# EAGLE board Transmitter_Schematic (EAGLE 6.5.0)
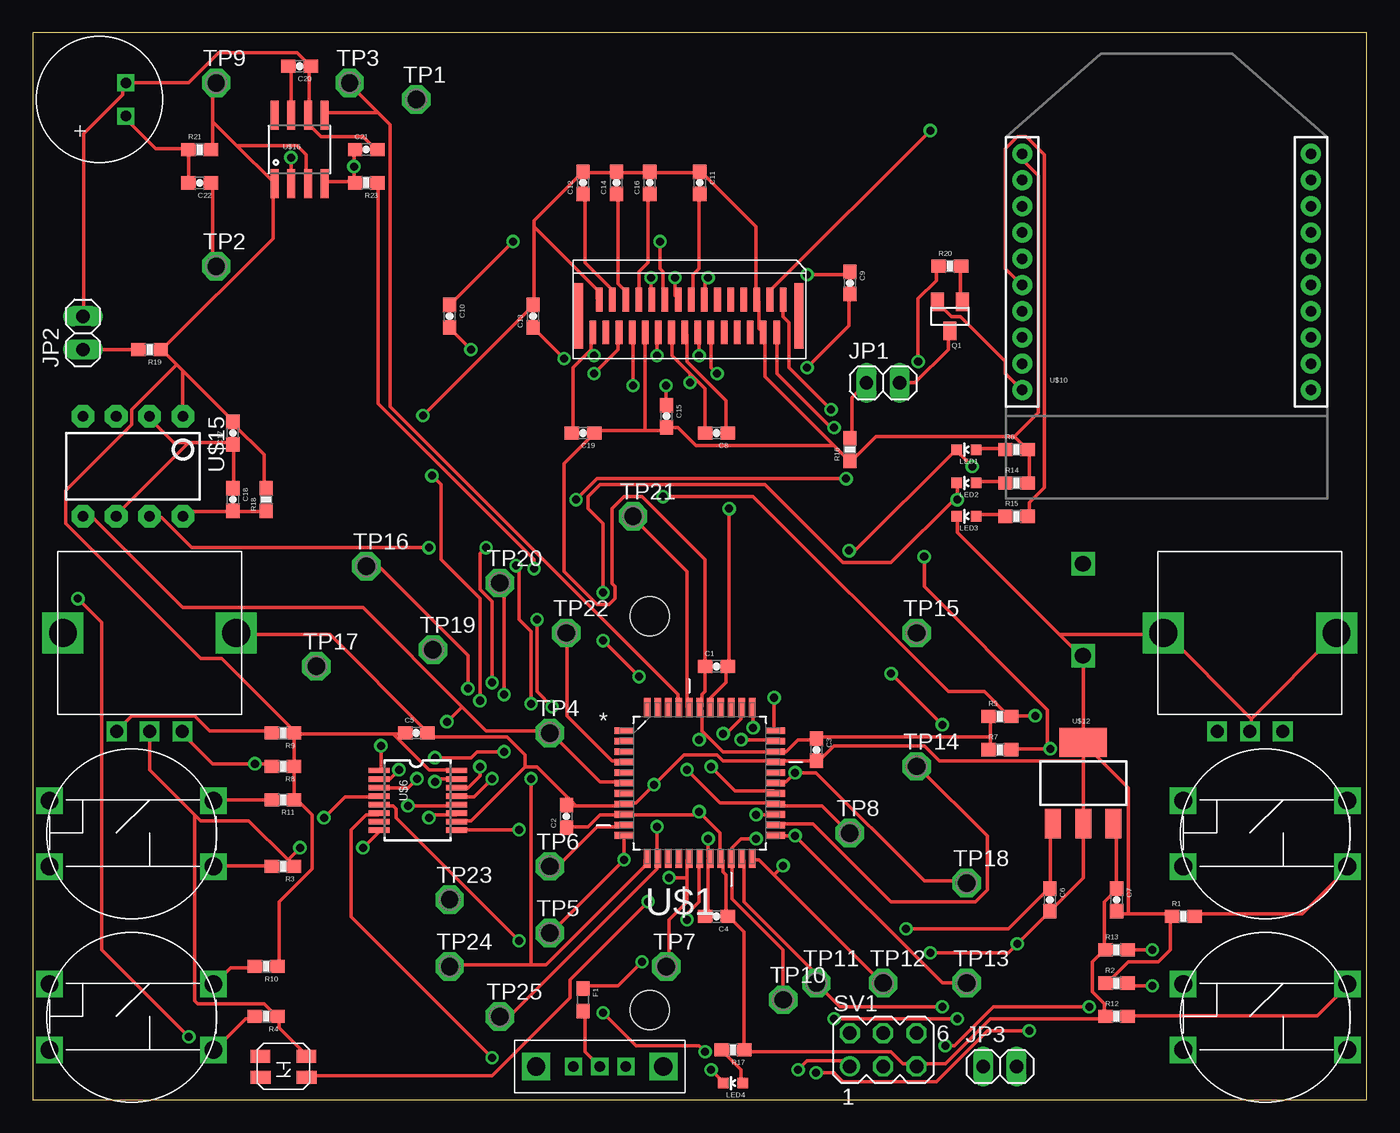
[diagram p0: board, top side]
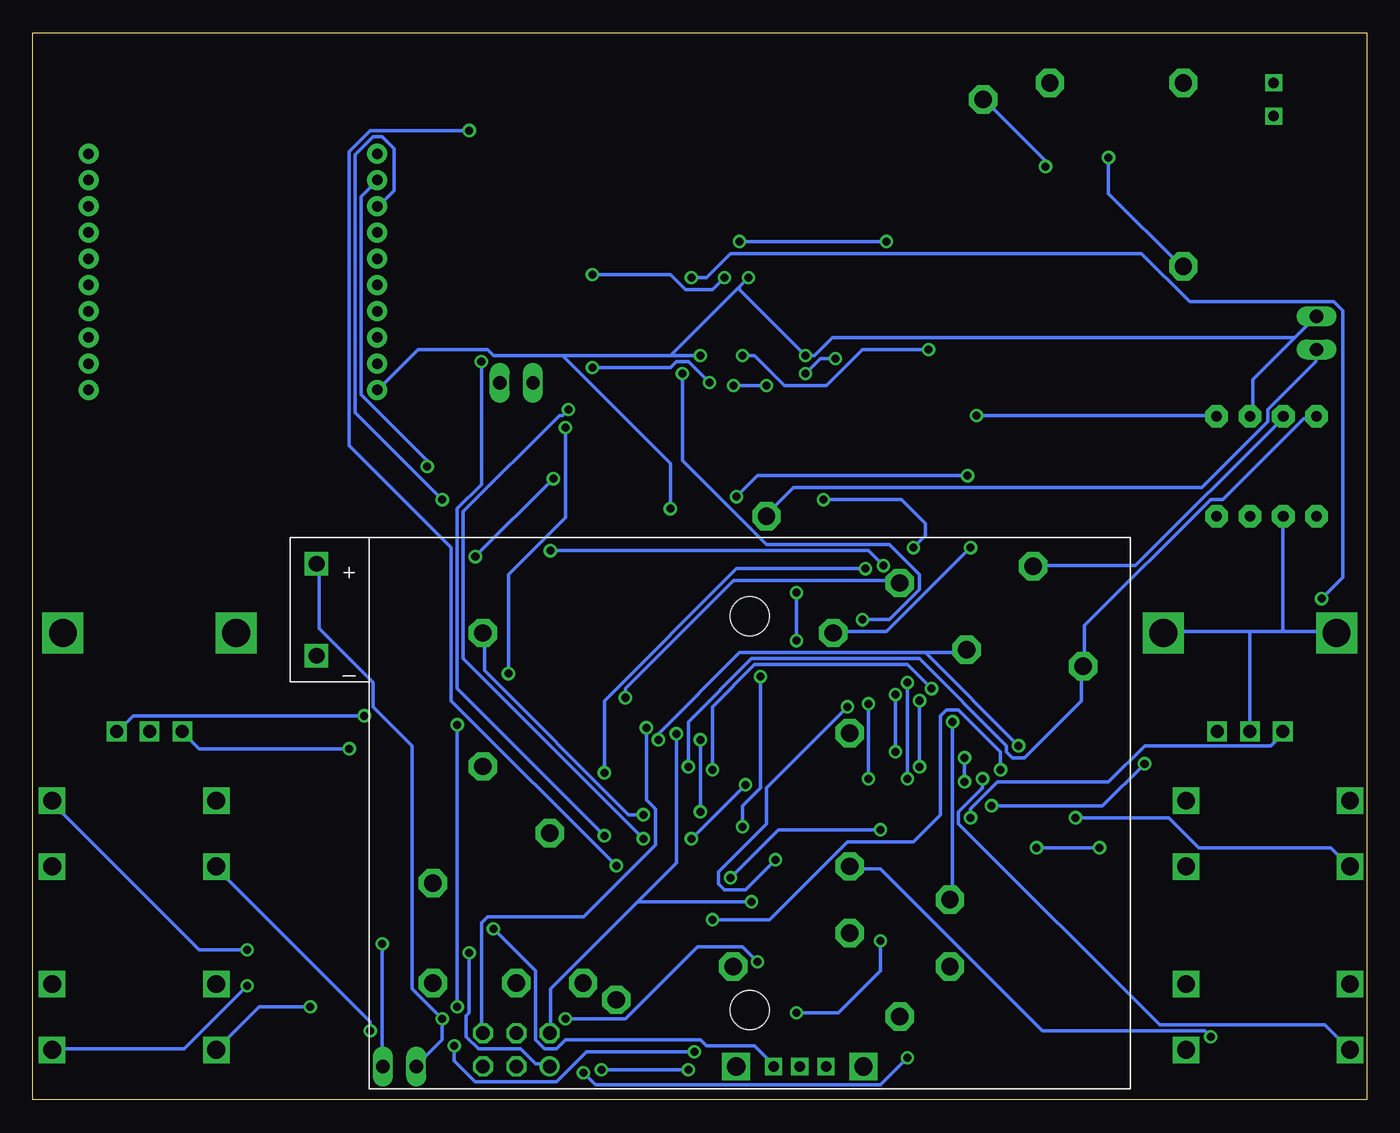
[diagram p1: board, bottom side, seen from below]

Size 101.6 x 81.28 mm. Coordinates in mm from the lower left corner, seen from the top.
Outline: 0,0 101.6,0 101.6,81.28 0,81.28 0,0
Copper layers (1*16): Top 0.035mm / dielectric 1.5mm / Bottom 0.035mm
Design rules "default": minimum track width 10mil, minimum drill 24mil, track to track 8mil, track to pad 8mil, pad to pad 8mil, via to via 8mil, smd to smd 8mil, copper to edge 40mil, drill to drill 8mil, minimum pad ring 10mil, minimum via ring 8mil, stop-mask expansion 4mil, vias tented up to drill 0mil, thermal gap 10mil

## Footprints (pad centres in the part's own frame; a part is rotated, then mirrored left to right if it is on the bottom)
0603-CAP = smd 1.1 x 1: 1 -0.85,0; 2 0.85,0
0603 = smd 1.1 x 1: 1 -0.85,0; 2 0.85,0
1X02 = drill 1.016 long: 1 -1.27,0; 2 1.27,0
LED-0603 = smd 0.8 x 0.8: A 0,-0.75; C 0,0.75
SOT23 = smd 1 x 1.4: 1 -0.95,-1.1; 2 0.95,-1.1; 3 0,1.1
0603-RES = smd 1.1 x 1: 1 -0.85,0; 2 0.85,0
MA03-2 = drill 1.016: 1 -2.54,-1.27 | drill 1.016 octagon: 2 -2.54,1.27; 3 0,-1.27; 4 0,1.27; 5 2.54,-1.27; 6 2.54,1.27
SPARKFUN_TAC_BUTTONS = drill 1.346 square: 1 0,5.004; 2 12.497,5.004; 3 0,0; 4 12.497,0
P1-13 = drill 1.321 pad 2.159 octagon: TP 0,0
QFP80P1200X1200X120-44N = smd 1.473 x 0.508: 1 -5.74,3.988; 2 -5.74,3.2; 3 -5.74,2.388; 4 -5.74,1.6; 5 -5.74,0.787; 6 -5.74,0; 7 -5.74,-0.787; 8 -5.74,-1.6; 9 -5.74,-2.388; 10 -5.74,-3.2; 11 -5.74,-3.988; 23 5.74,-3.988; 24 5.74,-3.2; 25 5.74,-2.388; 26 5.74,-1.6; 27 5.74,-0.787; 28 5.74,0; 29 5.74,0.787; 30 5.74,1.6; 31 5.74,2.388; 32 5.74,3.2; 33 5.74,3.988 | smd 0.508 x 1.473: 12 -3.988,-5.74; 13 -3.2,-5.74; 14 -2.388,-5.74; 15 -1.6,-5.74; 16 -0.787,-5.74; 17 0,-5.74; 18 0.787,-5.74; 19 1.6,-5.74; 20 2.388,-5.74; 21 3.2,-5.74; 22 3.988,-5.74; 34 3.988,5.74; 35 3.2,5.74; 36 2.388,5.74; 37 1.6,5.74; 38 0.787,5.74; 39 0,5.74; 40 -0.787,5.74; 41 -1.6,5.74; 42 -2.388,5.74; 43 -3.2,5.74; 44 -3.988,5.74
TSSOP16 = smd 0.4 x 1.6: 1 -2.225,-2.85; 2 -1.575,-2.85; 3 -0.925,-2.85; 4 -0.275,-2.85; 5 0.375,-2.85; 6 1.025,-2.85; 7 1.675,-2.85; 8 2.325,-2.85; 9 2.325,3.05; 10 1.675,3.05; 11 1.025,3.05; 12 0.375,3.05; 13 -0.275,3.05; 14 -0.925,3.05; 15 -1.575,3.05; 16 -2.225,3.05
MICRO_TAC_BUTTONS = smd 1.524 x 1: 1 0.75,2.1; 3 4.25,2.1 | smd 1.5 x 1: 2 0.75,0.5; 4 4.25,0.5
EVE_GE1F2012B = drill 2.1 square: @GND1 -6.6,0; @GND2 6.6,0 | drill 1 square: A -2.5,-7.5; B 2.5,-7.5; GND 0,-7.5
XBEE-1 = drill 0.8 pad 1.524: 1 -11,20; 2 -11,18; 3 -11,16; 4 -11,14; 5 -11,12; 6 -11,10; 7 -11,8; 8 -11,6; 9 -11,4; 10 -11,2; 11 11,2; 12 11,4; 13 11,6; 14 11,8; 15 11,10; 16 11,12; 17 11,14; 18 11,16; 19 11,18; 20 11,20
LCD_CONNECTOR = smd 0.5 x 1.8: 1 0,0; 2 -0.5,-2.5; 3 -1,0; 4 -1.5,-2.5; 5 -2,0; 6 -2.5,-2.5; 7 -3,0; 8 -3.5,-2.5; 9 -4,0; 10 -4.5,-2.5; 11 -5,0; 12 -5.5,-2.5; 13 -6,0; 14 -6.5,-2.5; 15 -7,0; 16 -7.5,-2.5; 17 -8,0; 18 -8.5,-2.5; 19 -9,0; 20 -9.5,-2.5; 21 -10,0; 22 -10.5,-2.5; 23 -11,0; 24 -11.5,-2.5; 25 -12,0; 26 -12.5,-2.5; 27 -13,0; 28 -13.5,-2.5; 29 -14,0; 30 -14.5,-2.5 | smd 0.7 x 5: 31 1.2,-1.25; 32 -15.6,-1.25
SOT223 = smd 1.219 x 2.235: 1 -2.311,-3.099; 2 0,-3.099; 3 2.311,-3.099 | smd 3.6 x 2.2: 4 0,3.099
3XAA_BATT_HOLDER = drill 1.2 square: + 33,-4; - 33,3 | hole 3: 0,30; 0,0
SWITCH_SLIDE = drill 0.8 square: 1 -2,0; 2 0,0; 3 2,0 | drill 1.41 square: P$4 4.85,0 | drill 1.4 square: P$5 -4.85,0
DIP08 = drill 0.813 pad 1.727 octagon: 1 -3.81,-3.81; 2 -1.27,-3.81; 3 1.27,-3.81; 4 3.81,-3.81; 5 3.81,3.81; 6 1.27,3.81; 7 -1.27,3.81; 8 -3.81,3.81
SOIC8 = smd 0.61 x 2.21: 1 -1.905,-2.616; 2 -0.635,-2.616; 3 0.635,-2.616; 4 1.905,-2.616; 5 1.905,2.616; 6 0.635,2.616; 7 -0.635,2.616; 8 -1.905,2.616
CMA-4544PF = drill 0.8 square: GND 2,1.27; OUT 2,-1.27

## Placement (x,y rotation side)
C1  0.1uF  [0603-CAP]  52.07,33.02 0 top
C2  0.1uF  [0603-CAP]  40.64,21.59 90 top
C3  0.1uF  [0603-CAP]  59.69,26.67 270 top
C4  0.1uF  [0603-CAP]  52.07,13.97 180 top
C5  0.1uF  [0603-CAP]  29.21,27.94 0 top
C6  0.1uF  [0603-CAP]  77.47,15.24 270 top
C7  10uF  [0603-CAP]  82.55,15.24 270 top
C8  0.1uF  [0603-CAP]  52.07,50.8 180 top
C9  0.1uF  [0603-CAP]  62.23,62.23 270 top
C10  0.1uF  [0603-CAP]  31.75,59.69 270 top
C11  0.1uF  [0603-CAP]  50.8,69.85 270 top
C12  0.1uF  [0603-CAP]  41.91,69.85 90 top
C13  0.1uF  [0603-CAP]  38.1,59.69 90 top
C14  0.1uF  [0603-CAP]  44.45,69.85 90 top
C15  0.1uF  [0603-CAP]  48.26,52.07 270 top
C16  0.1uF  [0603-CAP]  46.99,69.85 90 top
C17  0.1uF  [0603-CAP]  15.24,50.8 90 top
C18  0.33pF  [0603-CAP]  15.24,45.72 270 top
C19  0.1uF  [0603-CAP]  41.91,50.8 180 top
C20  0.1uF  [0603-CAP]  20.32,78.74 180 top
C21  0.1uF  [0603-CAP]  25.4,72.39 0 top
C22  0.1uF  [0603-CAP]  12.7,69.85 180 top
F1  PTC0603  [0603]  41.91,7.62 270 top
JP1  [1X02]  64.77,54.61 0 top
JP2  [1X02]  3.81,58.42 90 top
JP3  [1X02]  73.66,2.54 0 top
LED1  [LED-0603]  71.12,49.53 90 top
LED2  [LED-0603]  71.12,46.99 90 top
LED3  [LED-0603]  71.12,44.45 90 top
LED4  [LED-0603]  53.34,1.27 90 top
Q1  MMBT5088  [SOT23]  69.85,59.69 180 top
R1  10K  [0603-RES]  87.63,13.97 0 top
R2  10K  [0603-RES]  82.55,8.89 0 top
R3  10K  [0603-RES]  19.05,17.78 180 top
R4  10K  [0603-RES]  17.78,6.35 180 top
R5  10K  [0603-RES]  73.66,29.21 0 top
R6  1K  [0603-RES]  74.93,49.53 0 top
R7  10K  [0603-RES]  73.66,26.67 0 top
R8  10K  [0603-RES]  19.05,25.4 180 top
R9  10K  [0603-RES]  19.05,27.94 180 top
R10  4.7K  [0603-RES]  17.78,10.16 180 top
R11  4.7K  [0603-RES]  19.05,22.86 180 top
R12  4.7K  [0603-RES]  82.55,6.35 0 top
R13  4.7K  [0603-RES]  82.55,11.43 0 top
R14  1K  [0603-RES]  74.93,46.99 0 top
R15  1K  [0603-RES]  74.93,44.45 0 top
R16  100  [0603-RES]  62.23,49.53 90 top
R17  1.5K  [0603-RES]  53.34,3.81 180 top
R18  200K  [0603-RES]  17.78,45.72 90 top
R19  10K  [0603-RES]  8.89,57.15 180 top
R20  100  [0603-RES]  69.85,63.5 0 top
R21  100  [0603-RES]  12.7,72.39 0 top
R23  100  [0603-RES]  25.4,69.85 180 top
SV1  [MA03-2]  64.77,3.81 0 top
SW0  SPARKFUN_TAC_BUTTONS  [SPARKFUN_TAC_BUTTONS]  1.27,3.81 0 top
SW1  SPARKFUN_TAC_BUTTONS  [SPARKFUN_TAC_BUTTONS]  1.27,17.78 0 top
SW2  SPARKFUN_TAC_BUTTONS  [SPARKFUN_TAC_BUTTONS]  87.63,3.81 0 top
SW3  SPARKFUN_TAC_BUTTONS  [SPARKFUN_TAC_BUTTONS]  87.63,17.78 0 top
TP1  TPPAD1-13  [P1-13]  29.21,76.2 0 top
TP2  TPPAD1-13  [P1-13]  13.97,63.5 0 top
TP3  TPPAD1-13  [P1-13]  24.13,77.47 0 top
TP4  TPPAD1-13  [P1-13]  39.37,27.94 0 top
TP5  TPPAD1-13  [P1-13]  39.37,12.7 0 top
TP6  TPPAD1-13  [P1-13]  39.37,17.78 0 top
TP7  TPPAD1-13  [P1-13]  48.26,10.16 0 top
TP8  TPPAD1-13  [P1-13]  62.23,20.32 0 top
TP9  TPPAD1-13  [P1-13]  13.97,77.47 0 top
TP10  TPPAD1-13  [P1-13]  57.15,7.62 0 top
TP11  TPPAD1-13  [P1-13]  59.69,8.89 0 top
TP12  TPPAD1-13  [P1-13]  64.77,8.89 0 top
TP13  TPPAD1-13  [P1-13]  71.12,8.89 0 top
TP14  TPPAD1-13  [P1-13]  67.31,25.4 0 top
TP15  TPPAD1-13  [P1-13]  67.31,35.56 0 top
TP16  TPPAD1-13  [P1-13]  25.4,40.64 0 top
TP17  TPPAD1-13  [P1-13]  21.59,33.02 0 top
TP18  TPPAD1-13  [P1-13]  71.12,16.51 0 top
TP19  TPPAD1-13  [P1-13]  30.48,34.29 0 top
TP20  TPPAD1-13  [P1-13]  35.56,39.37 0 top
TP21  TPPAD1-13  [P1-13]  45.72,44.45 0 top
TP22  TPPAD1-13  [P1-13]  40.64,35.56 0 top
TP23  TPPAD1-13  [P1-13]  31.75,15.24 0 top
TP24  TPPAD1-13  [P1-13]  31.75,10.16 0 top
TP25  TPPAD1-13  [P1-13]  35.56,6.35 0 top
U$1  ATXMEGA32A4UTQFP44  [QFP80P1200X1200X120-44N]  50.8,24.13 0 top
U$6  8B_SHIFT_REG  [TSSOP16]  29.21,22.86 270 top
U$7  MICRO_TAC_BUTTONS  [MICRO_TAC_BUTTONS]  21.59,3.81 180 top
U$8  ENCODER  [EVE_GE1F2012B]  8.89,35.56 0 top
U$9  ENCODER  [EVE_GE1F2012B]  92.71,35.56 0 top
U$10  XBEE-1B1  [XBEE-1]  86.36,52.07 0 top
U$11  LCD_CONNECTOR  [LCD_CONNECTOR]  57.15,60.96 0 top
U$12  3.3V_REG_LDO  [SOT223]  80.01,24.13 0 top
U$13  3XAA_BATT_HOLDER  [3XAA_BATT_HOLDER]  46.99,36.83 180 bottom
U$14  SWITCH_SLIDE  [SWITCH_SLIDE]  43.18,2.54 0 top
U$15  FREQUENCY_DIVIDER  [DIP08]  7.62,48.26 180 top
U$16  LM4875  [SOIC8]  20.32,72.39 0 top
U$17  MICROPHONE  [CMA-4544PF]  5.08,76.2 0 top

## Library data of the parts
C1-C22 = SparkFun-Capacitors
F1 = SparkFun-PowerIC
JP1-JP3 = pinhead
LED1-LED4 = SparkFun-LED
Q1 = SparkFun-DiscreteSemi; PROD_ID: TRANS-11160
R1-R21 R23 = SparkFun-Resistors
SV1 = con-lstb; OC_FARNELL: unknown; OC_NEWARK: unknown
SW0 SW1-SW3 U$1 U$6-U$9 U$11-U$17 = TuansLib
TP1-TP25 = testpad
U$10 = SparkFun-RF

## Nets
3.3V: C1.1 C2.1 C3.1 C4.1 C5.1 C7.1 C11.1 C12.2 C13.2 C14.2 C15.2 C16.2 C17.2 C19.1 R5.1 R6.2 R7.1 R8.1 R9.1 R10.1 R11.1 R12.1 R13.1 R14.2 R16.1 R17.1 R18.2 R19.1 R21.2 SV1.5 TP9.TP U$1.9 U$1.19 U$1.31 U$1.39 U$6.16 U$10.1 U$11.4 U$11.5 U$11.22 U$11.29 U$12.3 U$15.1 U$16.1 U$16.3
AUD_IN: TP3.TP U$1.41 U$16.5
AUD_VOL: R23.1 TP18.TP U$1.28
FQD_AUDIO: TP4.TP TP23.TP U$1.6 U$15.5
FQD_RST: TP22.TP U$1.4 U$15.7
GND: C1.2 C2.2 C3.2 C4.2 C5.2 C6.2 C7.2 C17.1 C18.1 C19.2 C20.1 C21.2 JP2.2 JP3.2 LED3.C LED4.C Q1.2 R1.1 R2.1 R3.1 R4.1 SV1.1 U$1.8 U$1.18 U$1.30 U$1.38 U$6.8 U$6.10 U$7.2 U$8.@GND1 U$8.@GND2 U$8.GND U$9.@GND1 U$9.@GND2 U$9.GND U$10.10 U$11.14 U$11.21 U$11.30 U$12.2 U$12.4 U$13.- U$15.2 U$15.6 U$16.6 U$17.GND
LCD_LIGHT: R20.1 TP13.TP U$1.23
LCD_RST: TP11.TP U$1.21 U$11.2
LCD_SIG-SEL: TP12.TP U$1.22 U$11.3
LCD_SS: TP10.TP U$1.20 U$11.1
MIC_IN: C22.1 TP2.TP U$16.2
N$1: R2.2 SW2.4
N$2: C6.1 U$12.1 U$14.3
N$4: C8.1 U$11.16
N$5: C8.2 C9.2 U$11.18
N$6: R3.2 SW1.4
N$7: R4.2 SW0.4
N$8: R1.2 SW3.4
N$9: R5.2 U$6.14 U$9.B
N$10: C9.1 U$11.17
N$11: R9.2 U$6.11 U$8.A
N$12: R8.2 U$6.12 U$8.B
N$13: R7.2 U$6.13 U$9.A
N$14: C10.2 U$11.20
N$15: R10.2 SW0.2
N$16: R11.2 SW1.2
N$17: R12.2 SW2.2
N$18: R13.2 SW3.2
N$19: C10.1 U$11.19
N$20: C12.1 U$11.27
N$21: C13.1 U$11.26
N$22: C14.1 U$11.25
N$23: C15.1 U$11.24
N$24: C16.1 U$11.23
N$25: JP1.1 R16.2
N$26: C11.2 U$11.15
N$27: JP1.2 Q1.3
N$28: F1.2 U$14.2
N$29: LED1.A R6.1
N$30: LED2.A R14.1
N$31: LED3.A R15.1
N$32: LED4.A R17.2
N$33: Q1.1 R20.2
N$34: C22.2 R21.1 U$17.OUT
N$35: C21.1 R23.2 TP1.TP U$16.4
N$37: C20.2 U$16.7
N$40: C18.2 R18.1 U$15.8
PDI: SV1.6 U$1.34
PWR_RAW: F1.1 JP3.1 U$13.+
RST/PDI_CLK: SV1.2 U$1.35 U$7.1
SHIFT_LATCH: TP20.TP U$1.33 U$6.15
SHIFT_LOAD: TP19.TP U$1.32 U$6.1
SPIC_MISO: TP7.TP U$1.16 U$6.9
SPIC_MOSI: U$1.15
SPIC_SCK: U$1.17 U$6.2
SPIC_SS: U$1.14
SPID_MISO: TP8.TP TP16.TP U$1.26 U$15.3
SPID_MOSI: TP15.TP U$1.25
SPID_SCK: TP17.TP U$1.27 U$15.4
SPID_SS: TP14.TP U$1.24
SW0: SW0.3 U$6.3
SW1: SW1.3 U$6.4
SW2: SW2.3 U$6.5
SW3: SW3.3 U$6.6
TEMP_SENSOR: JP2.1 R19.2 TP21.TP U$1.40
TWIC_SCL: TP5.TP U$1.11 U$11.12
TWIC_SDA: TP6.TP U$1.10 U$11.13
USART_RXC0: LED1.C TP24.TP U$1.12 U$10.2
USART_TXC0: LED2.C TP25.TP U$1.13 U$10.3
XBEE_RSSI: R15.2 U$10.6

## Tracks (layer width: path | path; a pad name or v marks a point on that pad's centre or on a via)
3.3V  (via drill 0.61)
  Top 0.254: 72.92,27.66 72.92,29.03 R5.1 | 72.92,27.66 72.92,26.75 R7.1 | 72.92,27.66 59.89,27.66 C3.1 59.66,27.43 58.29,27.43 57.38,26.52 U$1.31 52.58,26.52 51.21,27.89 | 51.21,27.89 50.98,28.12 50.98,29.72 U$1.39 50.98,29.95 50.98,30.86 51.21,31.09 51.21,32.92 C1.1 51.21,33.15 51.21,41.15 46.41,45.95 45.03,45.95 44.12,45.03 44.12,39.32 44.35,39.09 44.35,38.18 43.89,37.72 42.98,37.72 40.46,40.23 40.46,48.46 42.75,50.75 C19.1 42.98,50.98 46.63,50.98 | 81.61,11.43 80.7,10.52 80.7,8.23 81.61,7.32 81.61,6.4 R12.1 81.61,6.17 72.92,6.17 69.49,2.74 67.44,2.74 SV1.5 67.21,2.74 66.29,2.74 65.38,3.66 54.41,3.66 R17.1 54.18,3.89 54.18,12.8 53.03,13.95 C4.1 52.81,14.17 52.81,17.14 52.58,17.37 52.58,18.29 U$1.19 52.35,18.52 52.35,20.34 50.98,21.72 50.75,21.72 | U$12.3 82.53,21.03 82.53,16.23 C7.1 82.53,16 81.61,15.09 81.61,11.43 | 81.61,11.43 R13.1 | C2.1 40.69,20.8 42.29,20.8 43.2,21.72 45.03,21.72 U$1.9 45.26,21.72 50.75,21.72 | v50.75,27.43 51.21,27.89 | 50.75,21.72 v50.75,21.95 | 38.18,66.52 38.18,66.98 41.83,70.64 C12.2 42.06,70.64 44.35,70.64 C14.2 44.58,70.64 46.86,70.64 C16.2 47.09,70.64 50.75,70.64 C11.1 50.98,70.64 55.09,66.52 55.09,61.04 U$11.5 55.32,60.81 55.32,58.75 55.55,58.52 U$11.4 55.78,58.29 55.78,55.09 61.04,49.84 | 38.18,66.52 38.18,60.58 C13.2 37.95,60.35 v29.72,52.12 | 38.18,66.52 42.98,61.72 42.98,61.04 U$11.29 | 46.63,50.98 48.01,50.98 48.23,51.21 C15.2 48.46,51.21 49.15,51.21 50.52,49.84 61.04,49.84 | 46.63,50.98 46.63,58.29 U$11.22 | R14.2 75.89,47.09 75.89,49.38 R6.2 75.67,49.61 74.75,50.52 | 61.04,49.84 62.18,48.69 R16.1 62.41,48.69 64.24,50.52 74.75,50.52
  Top 0.254: 74.75,50.52 76.58,52.35 76.58,70.41 75.44,71.55 75.44,72.01 U$10.1 | R10.1 18.75,10.29 18.75,15.09 21.26,17.6 21.26,21.72 20.12,22.86 R11.1 19.89,22.86 19.89,25.38 R8.1 19.89,25.6 19.89,27.89 R9.1 | 27.43,27.89 20.12,27.89 R9.1 | 27.43,27.89 28.35,27.89 C5.1 | 27.43,27.89 30.18,25.15 32.23,25.15 U$6.16 | 11.43,55.55 15.32,51.66 C17.2 15.32,51.44 17.6,49.15 17.6,46.63 R18.2 | 11.43,55.55 10.97,56.01 | 10.97,56.01 9.83,57.15 | 11.43,55.55 U$15.1 | 13.72,74.52 13.72,77.04 13.95,77.27 TP9.TP | 13.72,74.52 13.72,72.47 R21.2 | 13.72,74.52 15.54,72.69 | 15.54,72.69 18.29,69.95 U$16.1 18.29,69.72 18.29,65.61 9.83,57.15 | 15.54,72.69 20.12,72.69 20.8,72.01 20.8,69.95 U$16.3 | 9.83,57.15 R19.1 | 10.97,56.01 7.54,52.58 7.54,51.44 2.52,46.41 2.52,43.89 12.8,33.6 14.4,33.6 19.89,28.12 R9.1
  Bottom 0.254: v50.75,21.95 v50.75,27.43 | v29.72,52.12 11.43,52.12 U$15.1
AUD_IN
  Top 0.254: 26.29,75.21 24.23,77.27 TP3.TP | 26.29,75.21 27.2,74.3 27.2,52.81 49.15,30.86 49.15,29.95 U$1.41 | 26.29,75.21 22.4,75.21 U$16.5
AUD_VOL  (via drill 0.61)
  Top 0.254: v38.18,40.46 38.18,41.15 26.29,53.03 26.29,69.72 R23.1 | U$1.28 56.69,24.23 57.38,24.23 v58.06,24.92 59.66,24.92 67.89,16.69 71.09,16.69 TP18.TP
  Bottom 0.254: v38.18,40.46 48.01,40.46 58.06,30.4 v58.06,24.92
FQD_AUDIO  (via drill 0.61)
  Top 0.254: U$1.6 45.03,24.23 43.2,24.23 39.55,27.89 TP4.TP 39.32,28.12 34.52,28.12 32.69,29.95 | 32.69,29.95 25.15,37.49 11.43,37.49 4.57,44.35 3.89,44.35 U$15.5 | 32.69,29.95 v31.55,28.8
  Bottom 0.254: v31.55,28.8 31.55,15.32 TP23.TP
FQD_RST  (via drill 0.61)
  Top 0.254: U$1.4 45.03,25.83 44.12,25.83 40.69,29.26 40.69,35.43 TP22.TP | v30.18,42.06 12.12,42.06 9.83,44.35 8.91,44.35 U$15.7
  Bottom 0.254: v30.18,42.06 36.58,35.66 40.46,35.66 TP22.TP
GND  (via drill 0.61)
  Top 0.254: v51.66,2.29 52.58,1.37 LED4.C | v58.29,2.29 58.98,2.97 61.95,2.97 62.18,2.74 SV1.1 | v68.35,11.2 74.3,11.2 v74.98,11.89 77.27,14.17 C6.2 77.5,14.4 80.01,16.92 U$12.2 80.01,25.83 | 92.81,29.03 92.81,28.12 U$9.GND | 92.81,29.03 99.21,35.43 U$9.@GND2 | R2.1 81.84,8.91 83.44,10.52 85.72,10.52 86.64,11.43 86.64,13.95 R1.1 86.64,14.17 83.44,14.17 | 83.44,14.17 82.75,14.17 C7.2 | 78.18,35.43 79.78,33.83 U$13.- 80.01,33.6 U$12.4 80.01,27.2 | 78.18,35.43 70.41,43.2 70.41,44.35 LED3.C | 83.44,14.17 83.44,23.77 80.01,27.2 | 78.18,35.43 85.95,35.43 U$9.@GND1 86.18,35.66 92.81,29.03 | 80.01,27.2 80.01,25.83 | 42.29,56.92 42.52,57.15 42.52,58.29 U$11.30 | 42.29,56.92 41.15,55.78 41.15,50.98 C19.2 | U$1.38 51.66,29.95 51.66,30.63 52.81,31.77 52.81,32.92 C1.2 53.03,33.15 v53.03,45.03 | Q1.2 69.04,60.58 69.95,59.66 70.64,59.66 74.07,56.24 74.07,55.32 75.21,54.18 U$10.10 | v50.75,56.69 50.75,58.29 U$11.14 | v47.09,62.64 47.09,61.04 U$11.21 | 42.29,56.92 42.52,56.92 v42.75,56.69 | C21.2 26.06,72.47 25.15,73.38 21.95,73.38 21.03,74.3 21.03,74.98 U$16.6 21.03,75.21 21.03,78.64 C20.1 21.03,78.87 20.12,79.78 14.17,79.78 11.89,77.5 7.09,77.5 U$17.GND 6.86,77.27 6.86,76.58 3.89,73.61 3.89,59.89 JP2.2 | C18.1 15.32,46.63 15.32,49.84 C17.1 15.09,50.06 11.89,50.06 | 11.89,50.06 10.74,50.06 8.91,51.89 U$15.2 | 11.89,50.06 6.4,44.58 U$15.6 | U$7.2 20.8,3.43 18.75,5.49 18.75,6.17 R4.1 18.52,6.4 17.6,7.32 12.57,7.32 12.34,7.54 12.34,21.72 | 19.43,18.29 16.46,21.26 12.8,21.26 12.34,21.72 | 19.43,18.29 19.89,17.83 R3.1 | 12.34,21.72 8.91,25.15 8.91,27.89 U$8.GND | v25.15,19.2 26.29,20.34 U$6.8
  Top 0.254: 19.43,18.29 v20.34,19.2 | C4.2 51.44,14.17 51.44,18.29 U$1.18 51.44,18.52 v51.44,19.89 | 41.38,22.4 45.03,22.4 U$1.8 45.26,22.63 45.95,22.63 v47.32,24 49.61,26.29 52.12,26.29 52.58,25.83 56.46,25.83 U$1.30 56.69,25.83 59.66,25.83 C3.2 59.89,25.83 61.04,26.98 67.89,26.98 69.04,25.83 80.01,25.83 | 41.38,22.4 40.69,22.4 C2.2 | 37.49,25.38 33.38,21.26 32.46,21.26 U$6.10 | 37.49,25.38 38.41,25.38 41.38,22.4 | U$8.@GND2 15.54,35.43 22.63,35.43 29.95,28.12 C5.2 30.18,27.89 30.4,27.66 36.12,27.66 37.49,26.29 37.49,25.38
  Bottom 0.254: v58.29,2.29 v51.66,2.29 | v74.98,11.89 74.98,2.74 JP3.2 | v68.35,11.2 68.35,6.63 68.58,6.4 68.58,4.8 67.67,3.89 64.47,3.89 63.32,2.74 62.41,2.74 SV1.1 | 61.27,56.69 66.52,56.69 66.98,57.15 72.24,57.15 75.21,54.18 U$10.10 | 61.27,56.69 53.03,56.69 | 53.03,56.69 v50.75,56.69 | 53.03,56.69 47.78,61.95 | 47.78,61.95 v47.09,62.64 | v53.03,45.03 53.03,48.46 61.27,56.69 | 47.78,61.95 47.78,61.72 v42.75,56.69 42.06,56.69 40.69,58.06 5.49,58.06 | 5.49,58.06 8.69,54.86 8.69,52.12 U$15.2 | 5.49,58.06 3.89,59.66 JP2.2 | v20.34,19.2 v25.15,19.2 | v47.32,24 v51.44,19.89 | 8.91,35.66 15.32,35.66 U$8.@GND2 | 8.91,35.66 6.4,35.66 | 6.4,35.66 2.52,35.66 U$8.@GND1 | 8.91,35.66 8.91,28.12 U$8.GND | 6.4,35.66 6.4,44.35 U$15.6
LCD_LIGHT  (via drill 0.61)
  Top 0.254: v67.44,56.24 67.44,61.04 68.81,62.41 68.81,63.32 R20.1 | U$1.23 56.69,20.12 v58.06,20.12 69.27,8.91 71.09,8.91 TP13.TP
  Bottom 0.254: v67.44,56.24 67.44,46.86 69.27,45.03 69.27,31.32 v58.06,20.12
LCD_RST  (via drill 0.61)
  Top 0.254: U$1.21 54.18,18.29 54.18,15.09 59.66,9.6 59.66,8.91 TP11.TP 61.49,7.09 v69.27,7.09 | v61.04,51.21 60.81,51.21 56.69,55.32 56.69,58.29 U$11.2 | v69.27,28.57 v65.38,32.46
  Bottom 0.254: v61.04,51.21 61.04,44.35 65.38,40.01 v65.38,32.46 | v69.27,7.09 v69.27,28.57
LCD_SIG-SEL  (via drill 0.61)
  Top 0.254: 56.46,17.14 64.69,8.91 TP12.TP | 56.46,17.14 55.32,18.29 54.86,18.29 U$1.22 | v68.35,73.84 56.24,61.72 56.24,61.04 U$11.3 | 56.46,17.14 v57.15,17.83
  Bottom 0.254: v68.35,73.84 75.89,73.84 77.5,72.24 77.5,49.84 69.72,42.06 69.72,30.4 v57.15,17.83
LCD_SS  (via drill 0.61)
  Top 0.254: TP10.TP 57.15,11.43 53.26,15.32 53.26,18.29 U$1.20 53.26,18.52 53.26,19.2 53.95,19.89 v55.09,19.89 | U$11.1 57.15,59.66 57.61,59.21 57.61,55.78 v60.81,52.58
  Bottom 0.254: v60.81,52.58 61.27,52.12 61.49,52.12 68.81,44.81 68.81,33.6 v55.09,19.89
MIC_IN  (via drill 0.61)
  Top 0.254: C22.1 13.72,69.72 13.72,63.78 13.95,63.55 TP2.TP | v19.66,71.78 19.66,69.95 U$16.2
  Bottom 0.254: v19.66,71.78 19.66,69.04 14.17,63.55 TP2.TP
N$1  (via drill 0.61)
  Top 0.254: v85.27,8.69 83.44,8.69 R2.2
  Bottom 0.254: v85.27,8.69 90.07,3.89 100.13,3.89 SW2.4
N$2  (via drill 0.61)
  Top 0.254: U$12.1 77.5,21.03 77.5,16.23 C6.1 77.27,16 74.3,13.03 v66.52,13.03
  Bottom 0.254: v66.52,13.03 63.32,9.83 63.32,4.57 62.64,3.89 61.72,3.89 61.04,4.57 50.75,4.57 50.29,4.12 46.63,4.12 45.26,2.74 U$14.3
N$4
  Top 0.254: C8.1 52.81,50.98 52.81,53.26 49.84,56.24 49.84,58.29 U$11.16
N$5  (via drill 0.61)
  Top 0.254: 50.06,55.32 48.69,56.69 48.69,58.29 U$11.18 | 50.06,55.32 51.21,54.18 51.21,50.98 C8.2 | v58.98,55.78 62.18,58.98 62.18,61.27 C9.2 | 50.06,55.32 v50.06,54.63
  Bottom 0.254: v58.98,55.78 53.03,55.78 52.58,56.24 51.66,56.24 v50.06,54.63
N$6
  Top 0.254: R3.2 18.06,17.83 13.95,17.83 SW1.4
N$7
  Top 0.254: R4.2 16.92,6.17 16.23,6.17 13.95,3.89 SW0.4
N$8
  Top 0.254: R1.2 88.7,14.17 96.7,14.17 100.13,17.6 SW3.4
N$9  (via drill 0.61)
  Top 0.254: v76.35,29.26 74.52,29.26 R5.2 74.3,29.26 72.47,31.09 69.72,31.09 54.86,45.95 v48.01,45.95 | v34.06,25.38 34.06,24.69 33.15,23.77 32.46,23.77 U$6.14 | v34.06,30.4 34.06,38.18 31.09,41.15 31.09,46.86 v30.4,47.55
  Bottom 0.254: v76.35,29.26 93.95,29.26 95.1,28.12 U$9.B | v34.06,30.4 v34.06,25.38 | v30.4,47.55 46.41,47.55 v48.01,45.95
N$10  (via drill 0.61)
  Top 0.254: v58.98,62.87 62.18,62.87 C9.1 | v48.92,62.64 48.92,61.27 49.15,61.04 U$11.17
  Bottom 0.254: v58.98,62.87 53.03,62.87 51.89,61.72 49.84,61.72 v48.92,62.64
N$11  (via drill 0.61)
  Top 0.254: R9.2 18.06,28.12 13.49,28.12 12.34,29.26 7.54,29.26 6.4,28.12 U$8.A | v30.18,21.49 30.4,21.72 32.23,21.72 U$6.11
  Bottom 0.254: v30.18,21.49 30.18,22.17 28.12,24.23 19.66,24.23 16.92,26.98 7.32,26.98 6.4,27.89 U$8.A
N$12  (via drill 0.61)
  Top 0.254: R8.2 18.06,25.6 v16.92,25.6 13.72,25.6 11.43,27.89 U$8.B | v28.57,22.4 32.23,22.4 U$6.12
  Bottom 0.254: v28.57,22.4 20.12,22.4 v16.92,25.6
N$13  (via drill 0.61)
  Top 0.254: 77.27,26.75 74.52,26.75 R7.2 | v34.98,24.46 33.6,23.09 32.46,23.09 U$6.13 | v34.98,31.77 34.98,37.95 34.06,38.86 34.06,41.6 v34.52,42.06 | v41.38,45.72 42.98,47.32 v61.95,47.32 | v67.89,41.38 67.89,39.09 77.27,29.72 77.27,26.75 | 77.27,26.75 v77.5,26.75
  Bottom 0.254: v77.5,26.75 88.92,26.75 90.07,27.89 U$9.A | v34.98,31.77 v34.98,24.46 | v34.52,42.06 33.6,42.98 33.6,43.89 35.43,45.72 v41.38,45.72 | v67.89,41.38 v61.95,47.32
N$14  (via drill 0.61)
  Top 0.254: v33.38,57.15 31.77,58.75 C10.2 | v47.55,56.69 47.55,58.29 U$11.20
  Bottom 0.254: v33.38,57.15 38.41,57.15 41.15,54.41 44.35,54.41 46.63,56.69 v47.55,56.69
N$15
  Top 0.254: R10.2 16.92,10.06 15.09,10.06 13.95,8.91 SW0.2
N$16
  Top 0.254: R11.2 13.95,22.86 SW1.2
N$17
  Top 0.254: R12.2 83.44,6.4 97.84,6.4 100.13,8.69 SW2.2
N$18  (via drill 0.61)
  Top 0.254: v85.27,11.43 R13.2
  Bottom 0.254: v85.27,11.43 88.92,11.43 100.13,22.63 SW3.2
N$19  (via drill 0.61)
  Top 0.254: v36.58,65.38 31.77,60.58 C10.1 | v47.78,65.38 47.78,63.32 48.01,63.09 48.01,61.04 U$11.19
  Bottom 0.254: v47.78,65.38 v36.58,65.38
N$20
  Top 0.254: C12.1 42.06,68.81 42.06,63.78 44.12,61.72 44.12,61.04 U$11.27
N$21  (via drill 0.61)
  Top 0.254: v40.46,56.46 38.18,58.75 C13.1 | v42.75,55.32 44.58,57.15 44.58,58.29 U$11.26
  Bottom 0.254: v40.46,56.46 41.6,56.46 v42.75,55.32
N$22
  Top 0.254: C14.1 44.58,68.81 44.58,62.18 45.03,61.72 45.03,61.04 U$11.25
N$23  (via drill 0.61)
  Top 0.254: v48.23,54.41 48.23,53.03 C15.1 | v45.72,54.41 45.72,58.29 U$11.24
  Bottom 0.254: v45.72,54.41 v48.23,54.41
N$24
  Top 0.254: C16.1 46.86,68.81 46.86,63.78 46.18,63.09 46.18,61.04 U$11.23
N$25
  Top 0.254: R16.2 62.41,50.52 62.41,53.49 63.32,54.41 JP1.1
N$26
  Top 0.254: C11.2 50.75,68.81 50.75,63.32 50.29,62.87 50.29,61.04 U$11.15
N$27
  Top 0.254: Q1.3 69.72,58.52 69.72,57.15 67.21,54.63 66.06,54.63 JP1.2
N$28
  Top 0.254: U$14.2 42.06,3.66 42.06,6.63 F1.2
N$29
  Top 0.254: LED1.A 72.01,49.61 74.07,49.61 R6.1
N$30
  Top 0.254: LED2.A 72.01,47.09 74.07,47.09 R14.1
N$31
  Top 0.254: LED3.A 72.01,44.58 74.07,44.58 R15.1
N$32
  Top 0.254: LED4.A 53.95,1.37 53.95,2.29 52.58,3.66 R17.2
N$33
  Top 0.254: R20.2 70.64,63.32 70.64,60.81 Q1.1
N$34
  Top 0.254: C22.2 11.89,69.95 11.89,72.24 R21.1 11.66,72.47 9.37,72.47 7.09,74.75 U$17.OUT
N$35  (via drill 0.61)
  Top 0.254: 24.46,69.95 22.4,69.95 U$16.4 | 24.46,69.95 v24.46,71.09 24.46,72.24 C21.1 | 24.46,69.95 R23.2
  Bottom 0.254: v24.46,71.09 24.46,71.55 29.03,76.12 TP1.TP
N$37
  Top 0.254: C20.2 19.66,78.64 19.66,75.21 U$16.7
N$40
  Top 0.254: R18.1 17.6,44.81 15.32,44.81 C18.2 15.09,44.81 11.66,44.81 11.43,44.58 U$15.8
PDI  (via drill 0.61)
  Top 0.254: v54.86,28.35 54.86,29.72 U$1.34
  Bottom 0.254: v54.86,28.35 54.86,22.86 54.18,22.17 54.18,19.43 59.66,13.95 66.98,13.95 67.44,13.49 67.44,5.26 SV1.6
PWR_RAW  (via drill 0.61)
  Top 0.254: v46.41,10.52 44.58,8.69 42.06,8.69 F1.1 | v70.41,6.17 v61.04,6.17
  Bottom 0.254: v46.41,10.52 47.55,11.66 50.98,11.66 56.46,6.17 v61.04,6.17 | JP3.1 72.24,2.74 70.41,4.57 v70.41,6.17 72.69,8.46 72.69,26.98 75.67,29.95 75.67,31.77 79.78,35.89 79.78,40.69 U$13.+
RST/PDI_CLK  (via drill 0.61)
  Top 0.254: v52.58,27.89 52.81,27.89 53.95,29.03 53.95,29.72 U$1.35 | v46.86,15.09 40.92,9.14 40.92,7.77 34.98,1.83 21.03,1.83 U$7.1
  Bottom 0.254: v52.58,27.89 52.58,18.06 55.55,15.09 | 55.55,15.09 62.18,8.46 62.18,5.26 SV1.2 | 55.55,15.09 v46.86,15.09
SHIFT_LATCH  (via drill 0.61)
  Top 0.254: v56.46,30.63 56.46,28.12 U$1.33 | v30.63,24.23 30.86,24.46 32.23,24.46 U$6.15 | v30.63,26.06 33.38,26.06 33.83,26.52 v35.89,26.52 | v35.89,30.86 35.89,39.09 35.66,39.32 TP20.TP
  Bottom 0.254: v56.46,30.63 56.46,31.32 48.23,39.55 35.66,39.55 TP20.TP | v30.63,26.06 v30.63,24.23 | v35.89,30.86 v35.89,26.52
SHIFT_LOAD  (via drill 0.61)
  Top 0.254: v53.95,27.43 56.46,27.43 U$1.32 | v26.52,26.98 26.52,25.15 U$6.1
  Bottom 0.254: v53.95,27.43 53.95,27.89 47.78,34.06 33.6,34.06 | 33.6,34.06 30.86,34.06 30.63,34.29 TP19.TP | 33.6,34.06 v26.52,26.98
SPIC_MISO  (via drill 0.61)
  Top 0.254: 49.84,16.92 49.84,15.09 48.46,13.72 48.46,10.29 TP7.TP | 49.84,16.92 49.84,18.29 U$1.16 | v37.03,20.57 32.46,20.57 U$6.9 | 49.84,16.92 v48.46,16.92
  Bottom 0.254: v37.03,20.57 44.81,20.57 v48.46,16.92
SPIC_SCK  (via drill 0.61)
  Top 0.254: v49.84,13.72 49.84,14.17 50.75,15.09 50.75,18.29 U$1.17 | v27.89,25.15 27.2,24.46 26.52,24.46 U$6.2
  Bottom 0.254: v49.84,13.72 45.49,13.72 39.55,19.66 34.52,19.66 32.46,21.72 32.46,29.26 32,29.72 31.09,29.72 27.89,26.52 v27.89,25.15
SPID_MISO  (via drill 0.61)
  Top 0.254: TP8.TP 62.18,20.34 60.12,22.4 56.69,22.4 U$1.26 56.46,22.63 52.35,22.63 v49.84,25.15 | v33.15,31.32 33.15,33.83 26.52,40.46 25.6,40.46 TP16.TP
  Bottom 0.254: U$15.3 6.4,51.89 17.6,40.69 25.38,40.69 TP16.TP | v49.84,25.15 49.84,29.95 46.63,33.15 34.98,33.15 v33.15,31.32
SPID_MOSI  (via drill 0.61)
  Top 0.254: v55.09,21.72 56.46,21.72 U$1.25
  Bottom 0.254: v55.09,21.72 56.24,21.72 67.21,32.69 67.21,35.43 TP15.TP
SPID_SCK  (via drill 0.61)
  Top 0.254: v51.66,25.38 53.49,23.55 56.46,23.55 U$1.27
  Bottom 0.254: v51.66,25.38 51.66,28.8 46.86,33.6 34.06,33.6 27.43,26.98 27.43,26.52 26.98,26.06 26.06,26.06 21.72,30.4 21.72,32.92 TP17.TP 21.49,33.15 21.49,36.12 11.89,45.72 10.97,45.72 4.8,51.89 3.89,51.89 U$15.4
SPID_SS
  Top 0.254: U$1.24 56.69,21.03 59.44,21.03 65.38,15.09 71.78,15.09 72.69,16 72.69,20.12 67.44,25.38 TP14.TP
SW0  (via drill 0.61)
  Top 0.254: v29.26,24.46 28.57,23.77 26.52,23.77 U$6.3
  Bottom 0.254: v29.26,24.46 29.26,23.77 31.09,21.95 31.09,21.03 15.77,5.71 3.2,5.71 1.37,3.89 SW0.3
SW1  (via drill 0.61)
  Top 0.254: v22.17,21.49 23.77,23.09 26.29,23.09 U$6.4
  Bottom 0.254: v22.17,21.49 15.09,21.49 12.8,19.2 2.74,19.2 1.37,17.83 SW1.3
SW2  (via drill 0.61)
  Top 0.254: v37.03,12.12 27.66,21.49 27.66,22.17 27.43,22.4 26.52,22.4 U$6.5 | v43.43,6.63 45.95,4.12 50.75,4.12 v51.21,3.66 | v69.49,4.12 70.18,4.12 73.15,7.09 v80.47,7.09
  Bottom 0.254: v37.03,12.12 37.03,9.83 40.23,6.63 v43.43,6.63 | v51.21,3.66 59.44,3.66 61.72,1.37 67.89,1.37 69.49,2.97 v69.49,4.12 | v80.47,7.09 84.35,7.09 SW2.3
SW3  (via drill 0.61)
  Top 0.254: v34.98,3.2 24.23,13.95 24.23,20.57 25.38,21.72 26.29,21.72 U$6.6 | v59.66,2.06 61.04,2.06 61.72,1.37 68.81,1.37 72.69,5.26 v75.89,5.26
  Bottom 0.254: v34.98,3.2 37.03,1.14 58.75,1.14 v59.66,2.06 | v75.89,5.26 75.89,5.94 87.55,17.6 SW3.3
TEMP_SENSOR
  Top 0.254: JP2.1 R19.2 | U$1.40 49.84,29.95 49.84,40.23 45.72,44.35 TP21.TP
  Bottom 0.254: JP2.1 3.89,57.15 3.89,56.24 7.54,52.58 7.54,51.66 12.57,46.63 43.66,46.63 45.72,44.58 TP21.TP
TWIC_SCL  (via drill 0.61)
  Top 0.254: U$1.11 45.03,20.12 v45.03,18.29 39.55,12.8 TP5.TP | v52.12,55.32 51.66,55.78 51.66,58.29 U$11.12 | v38.41,36.58 38.41,31.09 v39.55,29.95
  Bottom 0.254: v52.12,55.32 52.12,48.69 45.72,42.29 36.35,42.29 34.06,40.01 34.06,38.86 36.35,36.58 v38.41,36.58 | v39.55,29.95 45.72,23.77 45.72,21.03 49.38,17.37 49.38,16.46 48.92,16 47.32,16 v45.03,18.29
TWIC_SDA  (via drill 0.61)
  Top 0.254: U$1.10 45.03,20.8 42.98,20.8 40.01,17.83 39.55,17.83 TP6.TP | v51.44,62.64 51.21,62.41 51.21,61.04 U$11.13 | v3.43,38.18 5.26,36.35 5.26,11.43 v11.89,4.8
  Bottom 0.254: v51.44,62.64 50.29,62.64 48.46,64.47 17.14,64.47 13.49,60.81 2.52,60.81 1.83,60.12 1.83,39.78 v3.43,38.18 | v11.89,4.8 12.34,5.26 24.69,5.26 37.03,17.6 39.32,17.6 TP6.TP
USART_RXC0  (via drill 0.61)
  Top 0.254: 37.95,10.29 31.77,10.29 TP24.TP | 37.95,10.29 39.09,10.29 46.63,17.83 46.63,18.29 U$1.12 | v71.55,48.23 70.41,49.38 LED1.C 70.18,49.38 62.64,41.83 v62.18,41.83 | v37.95,24.46 37.95,10.29 | v37.95,30.18 37.95,35.66 37.03,36.58 37.03,40.46 v36.8,40.69
  Bottom 0.254: v71.55,48.23 71.55,48.69 76.58,53.72 76.58,68.81 75.44,69.95 U$10.2 | v37.95,30.18 v37.95,24.46 | v36.8,40.69 37.95,41.83 v62.18,41.83
USART_TXC0  (via drill 0.61)
  Top 0.254: TP25.TP 35.66,6.4 36.35,6.4 47.55,17.6 47.55,18.29 U$1.13 47.55,18.52 v47.55,20.8 | 70.41,45.95 70.41,46.86 LED2.C | v43.43,34.98 v46.18,32.23 | v43.43,38.63 43.43,43.89 42.29,45.03 42.29,45.95 43.2,46.86 55.78,46.86 61.72,40.92 65.38,40.92 70.41,45.95 | 70.41,45.95 v70.41,45.72
  Bottom 0.254: v70.41,45.72 77.04,52.35 77.04,72.01 75.67,73.38 74.98,73.38 74.07,72.47 74.07,69.27 75.21,68.12 U$10.3 | v47.55,20.8 47.55,22.4 46.18,23.77 v46.18,32.23 | v43.43,38.63 v43.43,34.98
XBEE_RSSI
  Top 0.254: R15.2 75.89,44.58 75.89,45.49 77.04,46.63 77.04,72.01 75.67,73.38 74.98,73.38 74.07,72.47 74.07,63.32 75.21,62.18 U$10.6

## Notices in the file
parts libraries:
SparkFun-Capacitors: Licensing: CC v3.0 Share-Alike You are welcome to use this library for commercial purposes.
